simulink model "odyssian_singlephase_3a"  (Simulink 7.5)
settings: Solver=ode23t  StartTime=0.0  StopTime=10  RelTol=1e-6
undefined symbols (not defined in the file or in its folder): dfilt, DiscIntNeverNeededParam
libraries: powerlib x61, powerlib_extras x25, simulink x12, dsparch4 x2
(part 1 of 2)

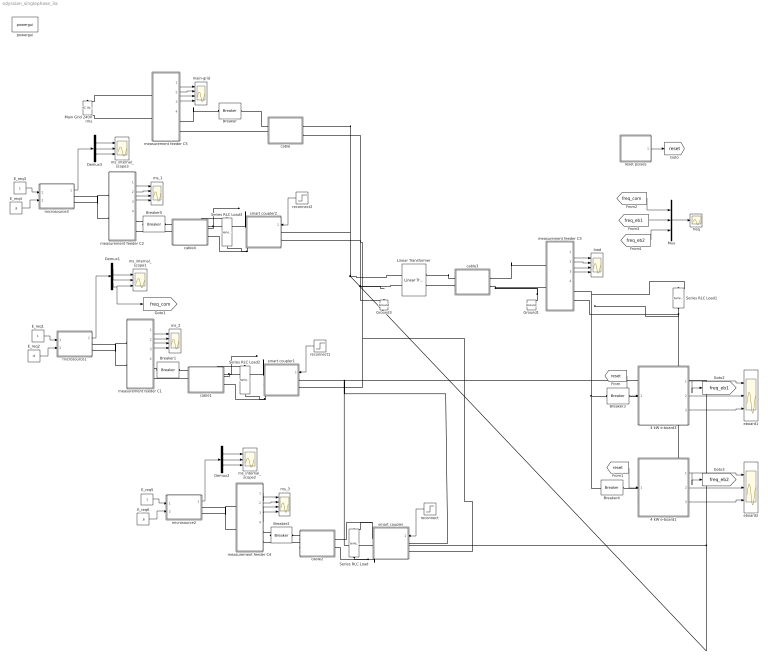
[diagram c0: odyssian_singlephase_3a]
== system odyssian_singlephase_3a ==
  " load" : Scope  NumInputPorts=4
  " main-grid" : Scope  NumInputPorts=4
  " ms_1" : Scope  NumInputPorts=4
  " ms_2" : Scope  NumInputPorts=4
  " ms_3" : Scope  NumInputPorts=4
  4 kW e-board1 : Subsystem  mask{tf=100, p=2}
      mask prompts: tf "fault_time"; p "load priority"
  4 kW e-board3 : Subsystem  mask{tf=100, p=2}
      mask prompts: tf "fault_time"; p "load priority"
  Breaker : powerlib/Elements/Breaker  DialogController=POWERSYS.PowerSysDialog  SystemSampleTime=-1  BreakerResistance=0.01  InitialState=1  SnubberResistance=1e6  SnubberCapacitance=inf  SwitchingTimes=[5]  External=off  Measurements=None  MoreParameters=off  NoBreakLoop=off
  Breaker{1..5} (5 alike) : powerlib/Elements/Breaker  DialogController=POWERSYS.PowerSysDialog  SystemSampleTime=-1  BreakerResistance=0.01  InitialState=1  SnubberResistance=1e6  SnubberCapacitance=inf  SwitchingTimes=[100]  External=off  Measurements=None  MoreParameters=off  NoBreakLoop=off
  Demux1 : Demux  Outputs=3
  Demux2 : Demux  Outputs=3
  Demux3 : Demux  Outputs=3
  E_req1 : Constant  OutDataType=fixdt(1, 16)  OutScaling=2^0
  E_req2 : Constant  Value=.8  OutDataType=fixdt(1, 16)  OutScaling=2^0
  E_req3 : Constant  OutDataType=fixdt(1, 16)  OutScaling=2^0
  E_req4 : Constant  Value=.8  OutDataType=fixdt(1, 16)  OutScaling=2^0
  E_req5 : Constant  OutDataType=fixdt(1, 16)  OutScaling=2^0
  E_req6 : Constant  Value=.8  OutDataType=fixdt(1, 16)  OutScaling=2^0
  Ground1 : powerlib/Elements/Ground  DialogController=POWERSYS.PowerSysDialog  PhysicalDomain=powersysdomain  SubClassName=unknown  LeftPortType=p1  RightPortType=p1  LConnTagsString=a
  Ground3 : powerlib/Elements/Ground  DialogController=POWERSYS.PowerSysDialog  PhysicalDomain=powersysdomain  SubClassName=unknown  LeftPortType=p1  RightPortType=p1  LConnTagsString=a
  Linear Transformer : powerlib/Elements/Linear Transformer  DialogController=POWERSYS.PowerSysDialog  PhysicalDomain=powersysdomain  SubClassName=unknown  LeftPortType=p1  RightPortType=p1  LConnTagsString=a|b  RConnTagsString=A|B  UNITS=SI  NominalPower=[ 45e3 , 60 ]  winding1=[240 0.001 1.e-5]  winding2=[120 .001 1.e-5]  ThreeWindings=off  winding3=[3.15e+05 0.7938 0.084225]  RmLm=[1.0804e+06 2866]  Measurements=All voltages and currents  DataType=on
  Main Grid 240V rms : powerlib/Electrical Sources/AC Voltage Source  DialogController=POWERSYS.PowerSysDialog  SystemSampleTime=-1  Amplitude=240*sqrt(2)  Phase=0  Frequency=60  SampleTime=0  Measurements=None
  Mux : Mux  Inputs=3
  Series RLC Load : powerlib/Elements/Series RLC Load  DialogController=POWERSYS.PowerSysDialog  PhysicalDomain=powersysdomain  SubClassName=unknown  LeftPortType=p1  RightPortType=p1  LConnTagsString=a  RConnTagsString=__new0  NominalVoltage=240  NominalFrequency=60  ActivePower=10  InductivePower=0  CapacitivePower=10*sin(acos(.88))  Setx0=off  InitialVoltage=0  SetiL0=off  InitialCurrent=0  Measurements=None
  Series RLC Load1 : powerlib/Elements/Series RLC Load  DialogController=POWERSYS.PowerSysDialog  PhysicalDomain=powersysdomain  SubClassName=unknown  LeftPortType=p1  RightPortType=p1  LConnTagsString=a  RConnTagsString=__new0  NominalVoltage=120  NominalFrequency=60  ActivePower=120  InductivePower=0  CapacitivePower=0  Setx0=off  InitialVoltage=0  SetiL0=off  InitialCurrent=0  Measurements=None
  Series RLC Load2 : powerlib/Elements/Series RLC Load  DialogController=POWERSYS.PowerSysDialog  PhysicalDomain=powersysdomain  SubClassName=unknown  LeftPortType=p1  RightPortType=p1  LConnTagsString=a  RConnTagsString=__new0  NominalVoltage=240  NominalFrequency=60  ActivePower=10  InductivePower=0  CapacitivePower=10*sin(acos(.88))  Setx0=off  InitialVoltage=0  SetiL0=off  InitialCurrent=0  Measurements=None
  Series RLC Load3 : powerlib/Elements/Series RLC Load  DialogController=POWERSYS.PowerSysDialog  PhysicalDomain=powersysdomain  SubClassName=unknown  LeftPortType=p1  RightPortType=p1  LConnTagsString=a  RConnTagsString=__new0  NominalVoltage=240  NominalFrequency=60  ActivePower=10  InductivePower=0  CapacitivePower=10*sin(acos(.88))  Setx0=off  InitialVoltage=0  SetiL0=off  InitialCurrent=0  Measurements=None
  cable : Subsystem
  cable1 : Subsystem
  cable2 : Subsystem
  cable3 : Subsystem
  cable4 : Subsystem
  eboard1 : Scope  NumInputPorts=3
  eboard2 : Scope  NumInputPorts=3
  freq : Scope
  measurement feeder C1 : Subsystem
  measurement feeder C2 : Subsystem
  measurement feeder C3 : Subsystem
  measurement feeder C4 : Subsystem
  measurement feeder C5 : Subsystem
  microsource1 : Subsystem  AncestorBlock=|
      | UWM_blocks/inverter-based
      | DG (simplified)
      | 208V - 15kVA
  microsource2 : Subsystem  AncestorBlock=|
      | UWM_blocks/inverter-based
      | DG (simplified)
      | 208V - 15kVA
  microsource3 : Subsystem  AncestorBlock=|
      | UWM_blocks/inverter-based
      | DG (simplified)
      | 208V - 15kVA
  ms_internal_scope1 : Scope  NumInputPorts=3
  ms_internal_scope2 : Scope  NumInputPorts=3
  ms_internal_scope3 : Scope  NumInputPorts=3
  powergui : powerlib/powergui  Priority=1  SystemSampleTime=-1  SimulationMode=Discrete  SampleTime=50e-5  frequency=60  SPID=off  DisableSnubberDevices=off  DisableRonSwitches=off  DisableVfSwitches=off  SwTol=0  Interpol=off  frequencyindice=0  echomessages=off  HookPort=off  DisplayEquations=off  FunctionMessages=off  EnableUseOfTLC=off  x0status=blocks  RestoreLinks=warning  ResistiveCurrentMeasurement=off  Frange=[0:2:500]  Ylog=off  Xlog=on  ShowGrid=off  save=off  variable=ZData  ZoomFFT=on  StartTime=0.0  cycles=1  DisplayStyle=1  fundamental=60  FreqAxis=off  MaxFrequency=1000  frequencyindicesteady=1  RmsSteady=1  display=off  Ts=0  methode=off
  reconnect : Step  Time=.1  SampleTime=0
  reconnect1 : Step  Time=.1  SampleTime=0
  reconnect2 : Step  Time=.1  SampleTime=0
  reset pulses : Subsystem  mask{tpulse=[50 100]}
  smart coupler : Subsystem
  smart coupler1 : Subsystem
  smart coupler2 : Subsystem
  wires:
  measurement feeder C3/1(Vm) -> " load"/1
  measurement feeder C3/2(Im) -> " load"/2
  measurement feeder C3/3(PQ) -> " load"/3
  measurement feeder C3/4(RMS (V-I)) -> " load"/4
  measurement feeder C4/1(Vm) -> " ms_3"/1
  measurement feeder C4/2(Im) -> " ms_3"/2
  measurement feeder C4/3(PQ) -> " ms_3"/3
  measurement feeder C4/4(RMS (V-I)) -> " ms_3"/4
  E_req6/1 -> microsource2/2(P_req)
  E_req5/1 -> microsource2/1(E_req)
  Demux2/2 -> ms_internal_scope2/2
  Demux2/1 -> ms_internal_scope2/1
  Demux2/3 -> ms_internal_scope2/3
  microsource2/1(m) -> Demux2/1
  reconnect/1 -> smart coupler/1(switch)
  4 kW e-board3/1(w) -> eboard1/1, [freq_eb1]
  4 kW e-board3/2(Irms) -> eboard1/2
  4 kW e-board3/3(Vrms) -> eboard1/3
  [reset] -> 4 kW e-board3/1(reset)
  4 kW e-board1/1(w) -> eboard2/1, [freq_eb2]
  4 kW e-board1/2(Irms) -> eboard2/2
  4 kW e-board1/3(Vrms) -> eboard2/3
  [reset] -> 4 kW e-board1/1(reset)
  Mux/1 -> freq/1
  reset pulses/1(Out1) -> [reset]
  [freq_com] -> Mux/1
  [freq_eb1] -> Mux/2
  [freq_eb2] -> Mux/3
  measurement feeder C5/1(Vm) -> " main-grid"/1
  measurement feeder C5/2(Im) -> " main-grid"/2
  measurement feeder C5/3(PQ) -> " main-grid"/3
  measurement feeder C5/4(RMS (V-I)) -> " main-grid"/4
  measurement feeder C1/1(Vm) -> " ms_2"/1
  measurement feeder C1/2(Im) -> " ms_2"/2
  measurement feeder C1/3(PQ) -> " ms_2"/3
  measurement feeder C1/4(RMS (V-I)) -> " ms_2"/4
  E_req2/1 -> microsource1/2(P_req)
  E_req1/1 -> microsource1/1(E_req)
  Demux1/2 -> ms_internal_scope1/2
  Demux1/1 -> ms_internal_scope1/1
  Demux1/3 -> ms_internal_scope1/3, [freq_com]
  microsource1/1(m) -> Demux1/1
  reconnect1/1 -> smart coupler1/1(switch)
  measurement feeder C2/1(Vm) -> " ms_1"/1
  measurement feeder C2/2(Im) -> " ms_1"/2
  measurement feeder C2/3(PQ) -> " ms_1"/3
  measurement feeder C2/4(RMS (V-I)) -> " ms_1"/4
  E_req4/1 -> microsource3/2(P_req)
  E_req3/1 -> microsource3/1(E_req)
  Demux3/2 -> ms_internal_scope3/2
  Demux3/1 -> ms_internal_scope3/1
  Demux3/3 -> ms_internal_scope3/3
  microsource3/1(m) -> Demux3/1
  reconnect2/1 -> smart coupler2/1(switch)
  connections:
  Breaker3/RConn1 -- measurement feeder C3/RConn1 -- Series RLC Load1/LConn1 -- Breaker4/RConn1
  Series RLC Load1/RConn1 -- measurement feeder C3/RConn2 -- 4 kW e-board3/LConn2 -- 4 kW e-board1/LConn2
  cable3/LConn2 -- Ground1/LConn1 -- measurement feeder C3/LConn2
  measurement feeder C4/LConn2 -- microsource2/RConn2
  measurement feeder C4/LConn1 -- microsource2/RConn1
  Breaker2/RConn1 -- measurement feeder C4/RConn1
  4 kW e-board3/LConn1 -- Breaker3/LConn1
  4 kW e-board1/LConn1 -- Breaker4/LConn1
  measurement feeder C5/RConn1 -- Breaker/LConn1
  cable/RConn2 -- measurement feeder C5/RConn2
  cable/RConn1 -- Breaker/RConn1
  Linear Transformer/LConn1 -- smart coupler/LConn1 -- smart coupler1/LConn1 -- cable/LConn1 -- smart coupler2/LConn1
  Linear Transformer/LConn2 -- Ground3/LConn1 -- smart coupler/LConn2 -- smart coupler1/LConn2 -- cable/LConn2 -- smart coupler2/LConn2
  cable2/RConn1 -- Breaker2/LConn1
  cable2/RConn2 -- measurement feeder C4/RConn2
  cable3/LConn1 -- measurement feeder C3/LConn1
  cable3/RConn2 -- Linear Transformer/RConn2
  cable3/RConn1 -- Linear Transformer/RConn1
  Series RLC Load/RConn1 -- cable2/LConn2 -- smart coupler/RConn2
  smart coupler/RConn1 -- Series RLC Load/LConn1 -- cable2/LConn1
  measurement feeder C5/LConn1 -- Main Grid 240V rms/RConn1
  measurement feeder C5/LConn2 -- Main Grid 240V rms/LConn1
  smart coupler1/RConn2 -- Series RLC Load2/RConn1 -- cable1/LConn2
  cable1/LConn1 -- smart coupler1/RConn1 -- Series RLC Load2/LConn1
  cable1/RConn2 -- measurement feeder C1/RConn2
  measurement feeder C1/LConn1 -- microsource1/RConn1
  cable1/RConn1 -- Breaker1/LConn1
  measurement feeder C1/LConn2 -- microsource1/RConn2
  Breaker1/RConn1 -- measurement feeder C1/RConn1
  smart coupler2/RConn2 -- Series RLC Load3/RConn1 -- cable4/LConn2
  cable4/LConn1 -- smart coupler2/RConn1 -- Series RLC Load3/LConn1
  measurement feeder C2/LConn1 -- microsource3/RConn1
  cable4/RConn2 -- measurement feeder C2/RConn2
  measurement feeder C2/LConn2 -- microsource3/RConn2
  Breaker5/RConn1 -- measurement feeder C2/RConn1
  cable4/RConn1 -- Breaker5/LConn1

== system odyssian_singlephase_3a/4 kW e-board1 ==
  reset : Inport
  Breaker : powerlib/Elements/Breaker  DialogController=POWERSYS.PowerSysDialog  SystemSampleTime=-1  BreakerResistance=0.01  InitialState=1  SnubberResistance=1e6  SnubberCapacitance=inf  SwitchingTimes="[ 1/60  5/60 ]"  External=on  Measurements=None  MoreParameters=off  NoBreakLoop=off
  Current Measurement : powerlib/Measurements/Current Measurement  DialogController=POWERSYS.PowerSysDialog  SystemSampleTime=-1  PhasorSimulation=off  OutputType=Complex  PSBequivalent=0
  Ground : powerlib/Elements/Ground  DialogController=POWERSYS.PowerSysDialog  PhysicalDomain=powersysdomain  SubClassName=unknown  LeftPortType=p1  RightPortType=p1  LConnTagsString=a
  Series RLC Load : powerlib/Elements/Series RLC Load  DialogController=POWERSYS.PowerSysDialog  PhysicalDomain=powersysdomain  SubClassName=unknown  LeftPortType=p1  RightPortType=p1  LConnTagsString=a  RConnTagsString=__new0  NominalVoltage=120  NominalFrequency=60  ActivePower=120  InductivePower=0  CapacitivePower=0  Setx0=off  InitialVoltage=0  SetiL0=off  InitialCurrent=0  Measurements=None
  Voltage  Measurement : powerlib/Measurements/Voltage Measurement  DialogController=POWERSYS.PowerSysDialog  SystemSampleTime=-1  PhasorSimulation=off  OutputType=Complex  PSBequivalent=0
  trip : Subsystem  mask{p=p}
      mask prompts: p "priority level"
  A : PMIOPort  Port=1  Side=Left
  C : PMIOPort  Port=2  Side=Left
  w : Outport  OutDataType=fixdt(1, 16)  OutScaling=2^0
  Irms : Outport  Port=2  OutDataType=fixdt(1, 16)  OutScaling=2^0
  Vrms : Outport  Port=3  OutDataType=fixdt(1, 16)  OutScaling=2^0
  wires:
  trip/1(w) -> w/1
  Current Measurement/1 -> trip/3(I)
  Voltage  Measurement/1 -> trip/2(V)
  reset/1 -> trip/1(Reset)
  trip/2(trip) -> Breaker/1
  trip/3(Irms) -> Irms/1
  trip/4(Vrms) -> Vrms/1
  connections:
  A/RConn1 -- Current Measurement/LConn1 -- Voltage  Measurement/LConn1
  Voltage  Measurement/LConn2 -- Ground/LConn1
  Current Measurement/RConn1 -- Breaker/LConn1
  Series RLC Load/LConn1 -- Breaker/RConn1
  Series RLC Load/RConn1 -- C/RConn1

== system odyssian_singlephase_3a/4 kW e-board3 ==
  reset : Inport
  Breaker : powerlib/Elements/Breaker  DialogController=POWERSYS.PowerSysDialog  SystemSampleTime=-1  BreakerResistance=0.01  InitialState=1  SnubberResistance=1e6  SnubberCapacitance=inf  SwitchingTimes="[ 1/60  5/60 ]"  External=on  Measurements=None  MoreParameters=off  NoBreakLoop=off
  Current Measurement : powerlib/Measurements/Current Measurement  DialogController=POWERSYS.PowerSysDialog  SystemSampleTime=-1  PhasorSimulation=off  OutputType=Complex  PSBequivalent=0
  Ground : powerlib/Elements/Ground  DialogController=POWERSYS.PowerSysDialog  PhysicalDomain=powersysdomain  SubClassName=unknown  LeftPortType=p1  RightPortType=p1  LConnTagsString=a
  Series RLC Load : powerlib/Elements/Series RLC Load  DialogController=POWERSYS.PowerSysDialog  PhysicalDomain=powersysdomain  SubClassName=unknown  LeftPortType=p1  RightPortType=p1  LConnTagsString=a  RConnTagsString=__new0  NominalVoltage=120  NominalFrequency=60  ActivePower=120  InductivePower=0  CapacitivePower=0  Setx0=off  InitialVoltage=0  SetiL0=off  InitialCurrent=0  Measurements=None
  Voltage  Measurement : powerlib/Measurements/Voltage Measurement  DialogController=POWERSYS.PowerSysDialog  SystemSampleTime=-1  PhasorSimulation=off  OutputType=Complex  PSBequivalent=0
  trip : Subsystem  mask{p=p}
      mask prompts: p "priority level"
  A : PMIOPort  Port=1  Side=Left
  C : PMIOPort  Port=2  Side=Left
  w : Outport  OutDataType=fixdt(1, 16)  OutScaling=2^0
  Irms : Outport  Port=2  OutDataType=fixdt(1, 16)  OutScaling=2^0
  Vrms : Outport  Port=3  OutDataType=fixdt(1, 16)  OutScaling=2^0
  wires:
  trip/1(w) -> w/1
  Current Measurement/1 -> trip/3(I)
  Voltage  Measurement/1 -> trip/2(V)
  reset/1 -> trip/1(Reset)
  trip/2(trip) -> Breaker/1
  trip/3(Irms) -> Irms/1
  trip/4(Vrms) -> Vrms/1
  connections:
  A/RConn1 -- Current Measurement/LConn1 -- Voltage  Measurement/LConn1
  Voltage  Measurement/LConn2 -- Ground/LConn1
  Current Measurement/RConn1 -- Breaker/LConn1
  Series RLC Load/LConn1 -- Breaker/RConn1
  Series RLC Load/RConn1 -- C/RConn1

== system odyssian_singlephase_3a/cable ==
  Series RLC Branch : powerlib/Elements/Series RLC Branch  DialogController=POWERSYS.PowerSysDialog  PhysicalDomain=powersysdomain  SubClassName=unknown  LeftPortType=p1  RightPortType=p1  LConnTagsString=__new0  RConnTagsString=__new0  BranchType=RL  Resistance=.001  Inductance=1.e-5  SetiL0=off  InitialCurrent=0  Capacitance=1e-6  Setx0=off  InitialVoltage=0  Measurements=None
  A : PMIOPort  Tag=PMCPort  Port=1  Side=Left
  A' : PMIOPort  Tag=PMCPort  Port=2  Side=Right
  B' : PMIOPort  Tag=PMCPort  Port=3  Side=Right
  B : PMIOPort  Tag=PMCPort  Port=4  Side=Left
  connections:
  A/RConn1 -- Series RLC Branch/LConn1
  A'/RConn1 -- Series RLC Branch/RConn1
  B/RConn1 -- B'/RConn1

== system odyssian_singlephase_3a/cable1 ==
  Series RLC Branch : powerlib/Elements/Series RLC Branch  DialogController=POWERSYS.PowerSysDialog  PhysicalDomain=powersysdomain  SubClassName=unknown  LeftPortType=p1  RightPortType=p1  LConnTagsString=__new0  RConnTagsString=__new0  BranchType=RL  Resistance=.001  Inductance=1.e-6  SetiL0=off  InitialCurrent=0  Capacitance=1e-6  Setx0=off  InitialVoltage=0  Measurements=None
  A : PMIOPort  Tag=PMCPort  Port=1  Side=Left
  A' : PMIOPort  Tag=PMCPort  Port=2  Side=Right
  B' : PMIOPort  Tag=PMCPort  Port=3  Side=Right
  B : PMIOPort  Tag=PMCPort  Port=4  Side=Left
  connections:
  A/RConn1 -- Series RLC Branch/LConn1
  Series RLC Branch/RConn1 -- A'/RConn1
  B/RConn1 -- B'/RConn1

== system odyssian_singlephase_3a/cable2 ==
  Series RLC Branch : powerlib/Elements/Series RLC Branch  DialogController=POWERSYS.PowerSysDialog  PhysicalDomain=powersysdomain  SubClassName=unknown  LeftPortType=p1  RightPortType=p1  LConnTagsString=__new0  RConnTagsString=__new0  BranchType=RL  Resistance=.001  Inductance=1.e-6  SetiL0=off  InitialCurrent=0  Capacitance=1e-6  Setx0=off  InitialVoltage=0  Measurements=None
  A : PMIOPort  Tag=PMCPort  Port=1  Side=Left
  A' : PMIOPort  Tag=PMCPort  Port=2  Side=Right
  B' : PMIOPort  Tag=PMCPort  Port=3  Side=Right
  B : PMIOPort  Tag=PMCPort  Port=4  Side=Left
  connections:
  A/RConn1 -- Series RLC Branch/LConn1
  Series RLC Branch/RConn1 -- A'/RConn1
  B/RConn1 -- B'/RConn1

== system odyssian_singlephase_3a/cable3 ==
  Series RLC Branch : powerlib/Elements/Series RLC Branch  DialogController=POWERSYS.PowerSysDialog  PhysicalDomain=powersysdomain  SubClassName=unknown  LeftPortType=p1  RightPortType=p1  LConnTagsString=__new0  RConnTagsString=__new0  BranchType=RL  Resistance=.001  Inductance=1.e-6  SetiL0=off  InitialCurrent=0  Capacitance=1e-6  Setx0=off  InitialVoltage=0  Measurements=None
  A : PMIOPort  Tag=PMCPort  Port=1  Side=Left
  A' : PMIOPort  Tag=PMCPort  Port=2  Side=Right
  B' : PMIOPort  Tag=PMCPort  Port=3  Side=Right
  B : PMIOPort  Tag=PMCPort  Port=4  Side=Left
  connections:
  A/RConn1 -- Series RLC Branch/LConn1
  Series RLC Branch/RConn1 -- A'/RConn1
  B/RConn1 -- B'/RConn1

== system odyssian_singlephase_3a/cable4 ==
  Series RLC Branch : powerlib/Elements/Series RLC Branch  DialogController=POWERSYS.PowerSysDialog  PhysicalDomain=powersysdomain  SubClassName=unknown  LeftPortType=p1  RightPortType=p1  LConnTagsString=__new0  RConnTagsString=__new0  BranchType=RL  Resistance=.001  Inductance=1.e-6  SetiL0=off  InitialCurrent=0  Capacitance=1e-6  Setx0=off  InitialVoltage=0  Measurements=None
  A : PMIOPort  Tag=PMCPort  Port=1  Side=Left
  A' : PMIOPort  Tag=PMCPort  Port=2  Side=Right
  B' : PMIOPort  Tag=PMCPort  Port=3  Side=Right
  B : PMIOPort  Tag=PMCPort  Port=4  Side=Left
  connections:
  A/RConn1 -- Series RLC Branch/LConn1
  Series RLC Branch/RConn1 -- A'/RConn1
  B/RConn1 -- B'/RConn1

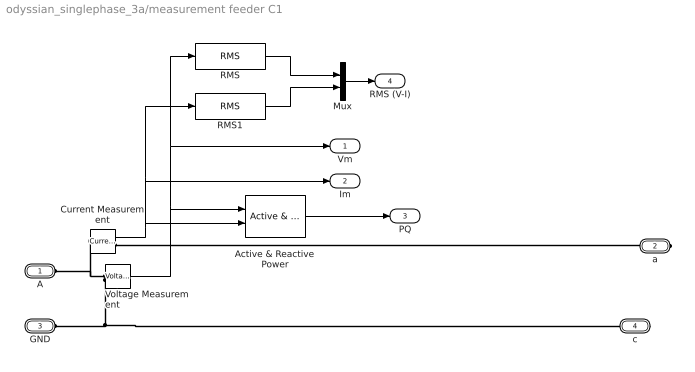
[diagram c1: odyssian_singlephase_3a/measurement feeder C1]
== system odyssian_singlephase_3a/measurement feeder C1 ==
  Active & Reactive Power : powerlib_extras/Measurements/Active & Reactive Power  DialogController=POWERSYS.PowerSysDialog  SystemSampleTime=-1  f1=60
  Current Measurement : powerlib/Measurements/Current Measurement  DialogController=POWERSYS.PowerSysDialog  SystemSampleTime=-1  PhasorSimulation=off  OutputType=Complex  PSBequivalent=0
  Mux : Mux  Inputs=2
  RMS : powerlib_extras/Measurements/RMS  DialogController=POWERSYS.PowerSysDialog  SystemSampleTime=-1  f1=60
  RMS1 : powerlib_extras/Measurements/RMS  DialogController=POWERSYS.PowerSysDialog  SystemSampleTime=-1  f1=60
  Voltage Measurement : powerlib/Measurements/Voltage Measurement  DialogController=POWERSYS.PowerSysDialog  SystemSampleTime=-1  PhasorSimulation=off  OutputType=Complex  PSBequivalent=0
  A : PMIOPort  Port=1  Side=Left
  a : PMIOPort  Port=2  Side=Right
  GND : PMIOPort  Port=3  Side=Left
  c : PMIOPort  Port=4  Side=Right
  Vm : Outport  OutDataType=fixdt(1, 16)  OutScaling=2^0
  Im : Outport  Port=2  OutDataType=fixdt(1, 16)  OutScaling=2^0
  PQ : Outport  Port=3  OutDataType=fixdt(1, 16)  OutScaling=2^0
  RMS (V-I) : Outport  Port=4  OutDataType=fixdt(1, 16)  OutScaling=2^0
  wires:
  Mux/1 -> RMS (V-I)/1
  Current Measurement/1 -> Im/1, RMS1/1, Active & Reactive Power/2
  Voltage Measurement/1 -> Vm/1, RMS/1, Active & Reactive Power/1
  Active & Reactive Power/1 -> PQ/1
  RMS/1 -> Mux/1
  RMS1/1 -> Mux/2
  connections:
  a/RConn1 -- Current Measurement/RConn1
  Voltage Measurement/LConn1 -- A/RConn1 -- Current Measurement/LConn1
  Voltage Measurement/LConn2 -- GND/RConn1 -- c/RConn1

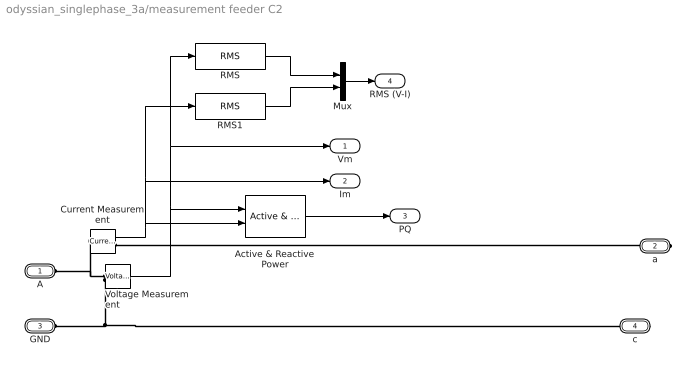
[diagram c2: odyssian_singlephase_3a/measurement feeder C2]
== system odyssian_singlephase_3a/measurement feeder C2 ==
  Active & Reactive Power : powerlib_extras/Measurements/Active & Reactive Power  DialogController=POWERSYS.PowerSysDialog  SystemSampleTime=-1  f1=60
  Current Measurement : powerlib/Measurements/Current Measurement  DialogController=POWERSYS.PowerSysDialog  SystemSampleTime=-1  PhasorSimulation=off  OutputType=Complex  PSBequivalent=0
  Mux : Mux  Inputs=2
  RMS : powerlib_extras/Measurements/RMS  DialogController=POWERSYS.PowerSysDialog  SystemSampleTime=-1  f1=60
  RMS1 : powerlib_extras/Measurements/RMS  DialogController=POWERSYS.PowerSysDialog  SystemSampleTime=-1  f1=60
  Voltage Measurement : powerlib/Measurements/Voltage Measurement  DialogController=POWERSYS.PowerSysDialog  SystemSampleTime=-1  PhasorSimulation=off  OutputType=Complex  PSBequivalent=0
  A : PMIOPort  Port=1  Side=Left
  a : PMIOPort  Port=2  Side=Right
  GND : PMIOPort  Port=3  Side=Left
  c : PMIOPort  Port=4  Side=Right
  Vm : Outport  OutDataType=fixdt(1, 16)  OutScaling=2^0
  Im : Outport  Port=2  OutDataType=fixdt(1, 16)  OutScaling=2^0
  PQ : Outport  Port=3  OutDataType=fixdt(1, 16)  OutScaling=2^0
  RMS (V-I) : Outport  Port=4  OutDataType=fixdt(1, 16)  OutScaling=2^0
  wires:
  Mux/1 -> RMS (V-I)/1
  Current Measurement/1 -> Im/1, RMS1/1, Active & Reactive Power/2
  Voltage Measurement/1 -> Vm/1, RMS/1, Active & Reactive Power/1
  Active & Reactive Power/1 -> PQ/1
  RMS/1 -> Mux/1
  RMS1/1 -> Mux/2
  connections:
  a/RConn1 -- Current Measurement/RConn1
  Voltage Measurement/LConn1 -- A/RConn1 -- Current Measurement/LConn1
  Voltage Measurement/LConn2 -- GND/RConn1 -- c/RConn1

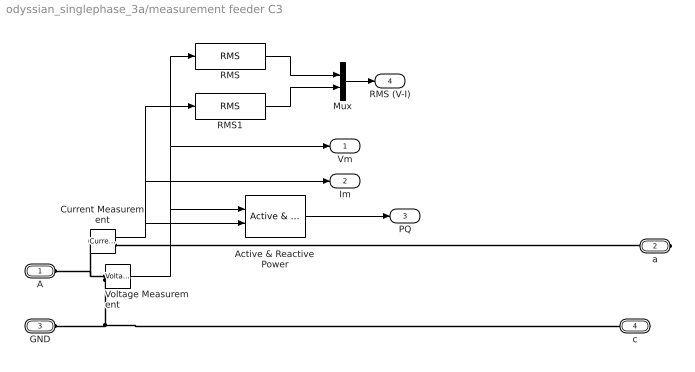
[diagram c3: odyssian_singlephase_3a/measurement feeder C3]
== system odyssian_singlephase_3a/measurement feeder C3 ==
  Active & Reactive Power : powerlib_extras/Measurements/Active & Reactive Power  DialogController=POWERSYS.PowerSysDialog  SystemSampleTime=-1  f1=60
  Current Measurement : powerlib/Measurements/Current Measurement  DialogController=POWERSYS.PowerSysDialog  SystemSampleTime=-1  PhasorSimulation=off  OutputType=Complex  PSBequivalent=0
  Mux : Mux  Inputs=2
  RMS : powerlib_extras/Measurements/RMS  DialogController=POWERSYS.PowerSysDialog  SystemSampleTime=-1  f1=60
  RMS1 : powerlib_extras/Measurements/RMS  DialogController=POWERSYS.PowerSysDialog  SystemSampleTime=-1  f1=60
  Voltage Measurement : powerlib/Measurements/Voltage Measurement  DialogController=POWERSYS.PowerSysDialog  SystemSampleTime=-1  PhasorSimulation=off  OutputType=Complex  PSBequivalent=0
  A : PMIOPort  Port=1  Side=Left
  a : PMIOPort  Port=2  Side=Right
  GND : PMIOPort  Port=3  Side=Left
  c : PMIOPort  Port=4  Side=Right
  Vm : Outport  OutDataType=fixdt(1, 16)  OutScaling=2^0
  Im : Outport  Port=2  OutDataType=fixdt(1, 16)  OutScaling=2^0
  PQ : Outport  Port=3  OutDataType=fixdt(1, 16)  OutScaling=2^0
  RMS (V-I) : Outport  Port=4  OutDataType=fixdt(1, 16)  OutScaling=2^0
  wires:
  Mux/1 -> RMS (V-I)/1
  Current Measurement/1 -> Im/1, RMS1/1, Active & Reactive Power/2
  Voltage Measurement/1 -> Vm/1, RMS/1, Active & Reactive Power/1
  Active & Reactive Power/1 -> PQ/1
  RMS/1 -> Mux/1
  RMS1/1 -> Mux/2
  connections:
  a/RConn1 -- Current Measurement/RConn1
  Voltage Measurement/LConn1 -- A/RConn1 -- Current Measurement/LConn1
  Voltage Measurement/LConn2 -- GND/RConn1 -- c/RConn1

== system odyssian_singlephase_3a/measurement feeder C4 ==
  Active & Reactive Power : powerlib_extras/Measurements/Active & Reactive Power  DialogController=POWERSYS.PowerSysDialog  SystemSampleTime=-1  f1=60
  Current Measurement : powerlib/Measurements/Current Measurement  DialogController=POWERSYS.PowerSysDialog  SystemSampleTime=-1  PhasorSimulation=off  OutputType=Complex  PSBequivalent=0
  Mux : Mux  Inputs=2
  RMS : powerlib_extras/Measurements/RMS  DialogController=POWERSYS.PowerSysDialog  SystemSampleTime=-1  f1=60
  RMS1 : powerlib_extras/Measurements/RMS  DialogController=POWERSYS.PowerSysDialog  SystemSampleTime=-1  f1=60
  Voltage Measurement : powerlib/Measurements/Voltage Measurement  DialogController=POWERSYS.PowerSysDialog  SystemSampleTime=-1  PhasorSimulation=off  OutputType=Complex  PSBequivalent=0
  A : PMIOPort  Port=1  Side=Left
  a : PMIOPort  Port=2  Side=Right
  GND : PMIOPort  Port=3  Side=Left
  c : PMIOPort  Port=4  Side=Right
  Vm : Outport  OutDataType=fixdt(1, 16)  OutScaling=2^0
  Im : Outport  Port=2  OutDataType=fixdt(1, 16)  OutScaling=2^0
  PQ : Outport  Port=3  OutDataType=fixdt(1, 16)  OutScaling=2^0
  RMS (V-I) : Outport  Port=4  OutDataType=fixdt(1, 16)  OutScaling=2^0
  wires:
  Mux/1 -> RMS (V-I)/1
  Current Measurement/1 -> Im/1, RMS1/1, Active & Reactive Power/2
  Voltage Measurement/1 -> Vm/1, RMS/1, Active & Reactive Power/1
  Active & Reactive Power/1 -> PQ/1
  RMS/1 -> Mux/1
  RMS1/1 -> Mux/2
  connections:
  a/RConn1 -- Current Measurement/RConn1
  Voltage Measurement/LConn1 -- A/RConn1 -- Current Measurement/LConn1
  Voltage Measurement/LConn2 -- GND/RConn1 -- c/RConn1

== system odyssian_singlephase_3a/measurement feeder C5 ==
  Active & Reactive Power : powerlib_extras/Measurements/Active & Reactive Power  DialogController=POWERSYS.PowerSysDialog  SystemSampleTime=-1  f1=60
  Current Measurement : powerlib/Measurements/Current Measurement  DialogController=POWERSYS.PowerSysDialog  SystemSampleTime=-1  PhasorSimulation=off  OutputType=Complex  PSBequivalent=0
  Mux : Mux  Inputs=2
  RMS : powerlib_extras/Measurements/RMS  DialogController=POWERSYS.PowerSysDialog  SystemSampleTime=-1  f1=60
  RMS1 : powerlib_extras/Measurements/RMS  DialogController=POWERSYS.PowerSysDialog  SystemSampleTime=-1  f1=60
  Voltage Measurement : powerlib/Measurements/Voltage Measurement  DialogController=POWERSYS.PowerSysDialog  SystemSampleTime=-1  PhasorSimulation=off  OutputType=Complex  PSBequivalent=0
  A : PMIOPort  Port=1  Side=Left
  a : PMIOPort  Port=2  Side=Right
  GND : PMIOPort  Port=3  Side=Left
  c : PMIOPort  Port=4  Side=Right
  Vm : Outport  OutDataType=fixdt(1, 16)  OutScaling=2^0
  Im : Outport  Port=2  OutDataType=fixdt(1, 16)  OutScaling=2^0
  PQ : Outport  Port=3  OutDataType=fixdt(1, 16)  OutScaling=2^0
  RMS (V-I) : Outport  Port=4  OutDataType=fixdt(1, 16)  OutScaling=2^0
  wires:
  Mux/1 -> RMS (V-I)/1
  Current Measurement/1 -> Im/1, RMS1/1, Active & Reactive Power/2
  Voltage Measurement/1 -> Vm/1, RMS/1, Active & Reactive Power/1
  Active & Reactive Power/1 -> PQ/1
  RMS/1 -> Mux/1
  RMS1/1 -> Mux/2
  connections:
  a/RConn1 -- Current Measurement/RConn1
  Voltage Measurement/LConn1 -- A/RConn1 -- Current Measurement/LConn1
  Voltage Measurement/LConn2 -- GND/RConn1 -- c/RConn1

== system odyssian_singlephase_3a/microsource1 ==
  E_req : Inport
  P_req : Inport  Port=2
  Current Measurement : powerlib/Measurements/Current Measurement  DialogController=POWERSYS.PowerSysDialog  SystemSampleTime=-1  PhasorSimulation=off  OutputType=Complex  PSBequivalent=0
  Gain : Gain  Gain=1/(2*pi)  ParameterDataType=fixdt(1, 16)  ParameterScaling=2^0  OutDataType=fixdt(1, 16)  OutScaling=2^0
  Linear Transformer : powerlib/Elements/Linear Transformer  DialogController=POWERSYS.PowerSysDialog  PhysicalDomain=powersysdomain  SubClassName=unknown  LeftPortType=p1  RightPortType=p1  LConnTagsString=a|b  RConnTagsString=A|B  UNITS=SI  NominalPower=[ 45e3 , 60 ]  winding1=[240 0.001 1.e-5]  winding2=[240 0.001 1.e-5]  ThreeWindings=off  winding3=[3.15e+05 0.7938 0.084225]  RmLm=[1.0804e+06 2866]  Measurements=All voltages and currents  DataType=on
  Mux : Mux  Inputs=3
  Parallel RLC Branch : powerlib/Elements/Parallel RLC Branch  DialogController=POWERSYS.PowerSysDialog  PhysicalDomain=powersysdomain  SubClassName=unknown  LeftPortType=p1  RightPortType=p1  LConnTagsString=a  RConnTagsString=__new0  BranchType=L  Resistance=1  Inductance=1.e-1  SetiL0=off  InitialCurrent=0  Capacitance=1e-6  Setx0=off  InitialVoltage=0  Measurements=None
  UWM_controller : Subsystem  mask{Vbase=240*sqrt(2), Sbase=200}
  Voltage Measurement : powerlib/Measurements/Voltage Measurement  DialogController=POWERSYS.PowerSysDialog  SystemSampleTime=-1  PhasorSimulation=off  OutputType=Complex  PSBequivalent=0
  microsource : Subsystem
  a : PMIOPort  Port=1  Side=Right
  GND : PMIOPort  Port=2  Side=Right
  m : Outport  OutDataType=fixdt(1, 16)  OutScaling=2^0
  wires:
  E_req/1 -> UWM_controller/3(E_req)
  P_req/1 -> UWM_controller/4(P_req)
  UWM_controller/1(Vpk) -> microsource/1(Vpk)
  UWM_controller/2(w) -> microsource/2(w), Gain/1
  Mux/1 -> m/1
  Gain/1 -> Mux/3
  Current Measurement/1 -> Mux/2, UWM_controller/2(i_meas)
  Voltage Measurement/1 -> Mux/1, UWM_controller/1(v_meas)
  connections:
  GND/RConn1 -- Voltage Measurement/LConn2 -- Linear Transformer/RConn2
  Linear Transformer/RConn1 -- Voltage Measurement/LConn1 -- Current Measurement/LConn1
  a/RConn1 -- Current Measurement/RConn1
  Parallel RLC Branch/LConn1 -- microsource/RConn1
  Linear Transformer/LConn1 -- Parallel RLC Branch/RConn1
  Linear Transformer/LConn2 -- microsource/RConn2

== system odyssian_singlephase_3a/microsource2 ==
  E_req : Inport
  P_req : Inport  Port=2
  Current Measurement : powerlib/Measurements/Current Measurement  DialogController=POWERSYS.PowerSysDialog  SystemSampleTime=-1  PhasorSimulation=off  OutputType=Complex  PSBequivalent=0
  Gain : Gain  Gain=1/(2*pi)  ParameterDataType=fixdt(1, 16)  ParameterScaling=2^0  OutDataType=fixdt(1, 16)  OutScaling=2^0
  Linear Transformer : powerlib/Elements/Linear Transformer  DialogController=POWERSYS.PowerSysDialog  PhysicalDomain=powersysdomain  SubClassName=unknown  LeftPortType=p1  RightPortType=p1  LConnTagsString=a|b  RConnTagsString=A|B  UNITS=SI  NominalPower=[ 45e3 , 60 ]  winding1=[240 0.001 1.e-5]  winding2=[240 0.001 1.e-5]  ThreeWindings=off  winding3=[3.15e+05 0.7938 0.084225]  RmLm=[1.0804e+06 2866]  Measurements=All voltages and currents  DataType=on
  Mux : Mux  Inputs=3
  Parallel RLC Branch : powerlib/Elements/Parallel RLC Branch  DialogController=POWERSYS.PowerSysDialog  PhysicalDomain=powersysdomain  SubClassName=unknown  LeftPortType=p1  RightPortType=p1  LConnTagsString=a  RConnTagsString=__new0  BranchType=L  Resistance=1  Inductance=1.e-1  SetiL0=off  InitialCurrent=0  Capacitance=1e-6  Setx0=off  InitialVoltage=0  Measurements=None
  UWM_controller : Subsystem  mask{Vbase=240*sqrt(2), Sbase=200}
  Voltage Measurement : powerlib/Measurements/Voltage Measurement  DialogController=POWERSYS.PowerSysDialog  SystemSampleTime=-1  PhasorSimulation=off  OutputType=Complex  PSBequivalent=0
  microsource : Subsystem
  a : PMIOPort  Port=1  Side=Right
  GND : PMIOPort  Port=2  Side=Right
  m : Outport  OutDataType=fixdt(1, 16)  OutScaling=2^0
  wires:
  E_req/1 -> UWM_controller/3(E_req)
  P_req/1 -> UWM_controller/4(P_req)
  UWM_controller/1(Vpk) -> microsource/1(Vpk)
  UWM_controller/2(w) -> microsource/2(w), Gain/1
  Mux/1 -> m/1
  Gain/1 -> Mux/3
  Current Measurement/1 -> Mux/2, UWM_controller/2(i_meas)
  Voltage Measurement/1 -> Mux/1, UWM_controller/1(v_meas)
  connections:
  GND/RConn1 -- Voltage Measurement/LConn2 -- Linear Transformer/RConn2
  Linear Transformer/RConn1 -- Voltage Measurement/LConn1 -- Current Measurement/LConn1
  a/RConn1 -- Current Measurement/RConn1
  Parallel RLC Branch/LConn1 -- microsource/RConn1
  Linear Transformer/LConn1 -- Parallel RLC Branch/RConn1
  Linear Transformer/LConn2 -- microsource/RConn2

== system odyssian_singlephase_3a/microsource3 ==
  E_req : Inport
  P_req : Inport  Port=2
  Current Measurement : powerlib/Measurements/Current Measurement  DialogController=POWERSYS.PowerSysDialog  SystemSampleTime=-1  PhasorSimulation=off  OutputType=Complex  PSBequivalent=0
  Gain : Gain  Gain=1/(2*pi)  ParameterDataType=fixdt(1, 16)  ParameterScaling=2^0  OutDataType=fixdt(1, 16)  OutScaling=2^0
  Linear Transformer : powerlib/Elements/Linear Transformer  DialogController=POWERSYS.PowerSysDialog  PhysicalDomain=powersysdomain  SubClassName=unknown  LeftPortType=p1  RightPortType=p1  LConnTagsString=a|b  RConnTagsString=A|B  UNITS=SI  NominalPower=[ 45e3 , 60 ]  winding1=[240 0.001 1.e-5]  winding2=[240 0.001 1.e-5]  ThreeWindings=off  winding3=[3.15e+05 0.7938 0.084225]  RmLm=[1.0804e+06 2866]  Measurements=All voltages and currents  DataType=on
  Mux : Mux  Inputs=3
  Parallel RLC Branch : powerlib/Elements/Parallel RLC Branch  DialogController=POWERSYS.PowerSysDialog  PhysicalDomain=powersysdomain  SubClassName=unknown  LeftPortType=p1  RightPortType=p1  LConnTagsString=a  RConnTagsString=__new0  BranchType=L  Resistance=1  Inductance=1.e-1  SetiL0=off  InitialCurrent=0  Capacitance=1e-6  Setx0=off  InitialVoltage=0  Measurements=None
  UWM_controller : Subsystem  mask{Vbase=240*sqrt(2), Sbase=200}
  Voltage Measurement : powerlib/Measurements/Voltage Measurement  DialogController=POWERSYS.PowerSysDialog  SystemSampleTime=-1  PhasorSimulation=off  OutputType=Complex  PSBequivalent=0
  microsource : Subsystem
  a : PMIOPort  Port=1  Side=Right
  GND : PMIOPort  Port=2  Side=Right
  m : Outport  OutDataType=fixdt(1, 16)  OutScaling=2^0
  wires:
  E_req/1 -> UWM_controller/3(E_req)
  P_req/1 -> UWM_controller/4(P_req)
  UWM_controller/1(Vpk) -> microsource/1(Vpk)
  UWM_controller/2(w) -> microsource/2(w), Gain/1
  Mux/1 -> m/1
  Gain/1 -> Mux/3
  Current Measurement/1 -> Mux/2, UWM_controller/2(i_meas)
  Voltage Measurement/1 -> Mux/1, UWM_controller/1(v_meas)
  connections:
  GND/RConn1 -- Voltage Measurement/LConn2 -- Linear Transformer/RConn2
  Linear Transformer/RConn1 -- Voltage Measurement/LConn1 -- Current Measurement/LConn1
  a/RConn1 -- Current Measurement/RConn1
  Parallel RLC Branch/LConn1 -- microsource/RConn1
  Linear Transformer/LConn1 -- Parallel RLC Branch/RConn1
  Linear Transformer/LConn2 -- microsource/RConn2

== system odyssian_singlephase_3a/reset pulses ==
  Sum : Sum  Inputs=|++  OutDataType=fixdt(1, 16)  OutScaling=2^0
  pulse : Subsystem  mask{tstart=tpulse(1), dt=.1}
  pulse1 : Subsystem  mask{tstart=tpulse(2), dt=.1}
  Out1 : Outport
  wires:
  pulse/1(Out1) -> Sum/1
  pulse1/1(Out1) -> Sum/2
  Sum/1 -> Out1/1

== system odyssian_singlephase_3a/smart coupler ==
  switch : Inport  OutDataType=fixdt(1, 16)  OutScaling=2^0
  Abs : Abs  OutDataType=fixdt(1, 16)  OutScaling=2^0
  Breaker : powerlib/Elements/Breaker  DialogController=POWERSYS.PowerSysDialog  SystemSampleTime=-1  BreakerResistance=0.01  InitialState=0  SnubberResistance=1e6  SnubberCapacitance=inf  SwitchingTimes="[ 1/60  5/60 ]"  External=on  Measurements=None  MoreParameters=off  NoBreakLoop=off
  Level-2 M-file S-Function : M-S-Function  FunctionName=smart_coupler
  Scope : Scope  NumInputPorts=3
  Transfer Fcn : TransferFcn  Numerator=[100]  Denominator=[1 100]
  Voltage Measurement : powerlib/Measurements/Voltage Measurement  DialogController=POWERSYS.PowerSysDialog  SystemSampleTime=-1  PhasorSimulation=off  OutputType=Complex  PSBequivalent=0
  A : PMIOPort  Port=1  Side=Left
  C : PMIOPort  Port=2  Side=Left
  a : PMIOPort  Port=3  Side=Right
  c : PMIOPort  Port=4  Side=Right
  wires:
  switch/1 -> Level-2 M-file S-Function/2, Scope/2
  Level-2 M-file S-Function/1 -> Scope/1, Breaker/1
  Voltage Measurement/1 -> Abs/1
  Abs/1 -> Transfer Fcn/1
  Transfer Fcn/1 -> Level-2 M-file S-Function/1, Scope/3
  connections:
  Breaker/LConn1 -- A/RConn1 -- Voltage Measurement/LConn1
  Breaker/RConn1 -- Voltage Measurement/LConn2 -- a/RConn1
  c/RConn1 -- C/RConn1

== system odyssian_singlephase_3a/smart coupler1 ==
  switch : Inport  OutDataType=fixdt(1, 16)  OutScaling=2^0
  Abs : Abs  OutDataType=fixdt(1, 16)  OutScaling=2^0
  Breaker : powerlib/Elements/Breaker  DialogController=POWERSYS.PowerSysDialog  SystemSampleTime=-1  BreakerResistance=0.01  InitialState=0  SnubberResistance=1e6  SnubberCapacitance=inf  SwitchingTimes="[ 1/60  5/60 ]"  External=on  Measurements=None  MoreParameters=off  NoBreakLoop=off
  Level-2 M-file S-Function : M-S-Function  FunctionName=smart_coupler
  Scope : Scope  NumInputPorts=3
  Transfer Fcn : TransferFcn  Numerator=[100]  Denominator=[1 100]
  Voltage Measurement : powerlib/Measurements/Voltage Measurement  DialogController=POWERSYS.PowerSysDialog  SystemSampleTime=-1  PhasorSimulation=off  OutputType=Complex  PSBequivalent=0
  A : PMIOPort  Port=1  Side=Left
  C : PMIOPort  Port=2  Side=Left
  a : PMIOPort  Port=3  Side=Right
  c : PMIOPort  Port=4  Side=Right
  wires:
  switch/1 -> Level-2 M-file S-Function/2, Scope/2
  Level-2 M-file S-Function/1 -> Scope/1, Breaker/1
  Voltage Measurement/1 -> Abs/1
  Abs/1 -> Transfer Fcn/1
  Transfer Fcn/1 -> Level-2 M-file S-Function/1, Scope/3
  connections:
  Breaker/LConn1 -- A/RConn1 -- Voltage Measurement/LConn1
  Breaker/RConn1 -- Voltage Measurement/LConn2 -- a/RConn1
  c/RConn1 -- C/RConn1

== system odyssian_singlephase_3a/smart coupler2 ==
  switch : Inport  OutDataType=fixdt(1, 16)  OutScaling=2^0
  Abs : Abs  OutDataType=fixdt(1, 16)  OutScaling=2^0
  Breaker : powerlib/Elements/Breaker  DialogController=POWERSYS.PowerSysDialog  SystemSampleTime=-1  BreakerResistance=0.01  InitialState=0  SnubberResistance=1e6  SnubberCapacitance=inf  SwitchingTimes="[ 1/60  5/60 ]"  External=on  Measurements=None  MoreParameters=off  NoBreakLoop=off
  Level-2 M-file S-Function : M-S-Function  FunctionName=smart_coupler
  Scope : Scope  NumInputPorts=3
  Transfer Fcn : TransferFcn  Numerator=[100]  Denominator=[1 100]
  Voltage Measurement : powerlib/Measurements/Voltage Measurement  DialogController=POWERSYS.PowerSysDialog  SystemSampleTime=-1  PhasorSimulation=off  OutputType=Complex  PSBequivalent=0
  A : PMIOPort  Port=1  Side=Left
  C : PMIOPort  Port=2  Side=Left
  a : PMIOPort  Port=3  Side=Right
  c : PMIOPort  Port=4  Side=Right
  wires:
  switch/1 -> Level-2 M-file S-Function/2, Scope/2
  Level-2 M-file S-Function/1 -> Scope/1, Breaker/1
  Voltage Measurement/1 -> Abs/1
  Abs/1 -> Transfer Fcn/1
  Transfer Fcn/1 -> Level-2 M-file S-Function/1, Scope/3
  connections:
  Breaker/LConn1 -- A/RConn1 -- Voltage Measurement/LConn1
  Breaker/RConn1 -- Voltage Measurement/LConn2 -- a/RConn1
  c/RConn1 -- C/RConn1

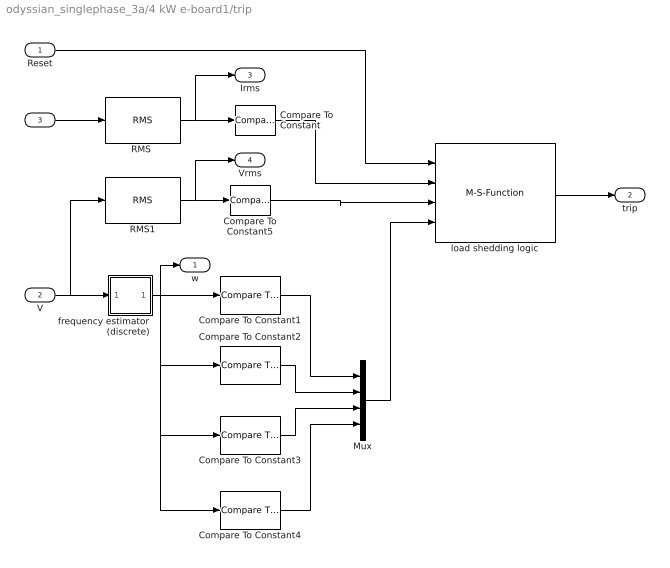
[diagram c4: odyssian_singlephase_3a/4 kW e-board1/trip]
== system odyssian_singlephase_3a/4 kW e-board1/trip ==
  Reset : Inport
  V : Inport  Port=2
  I : Inport  Port=3
  Compare To Constant : simulink/Logic and Bit Operations/Compare To Constant  SystemSampleTime=-1  relop=>=  const=100  LogicOutDataTypeMode=boolean
  Compare To Constant1 : simulink/Logic and Bit Operations/Compare To Constant  SystemSampleTime=-1  relop=<=  const=59.8  LogicOutDataTypeMode=boolean
  Compare To Constant2 : simulink/Logic and Bit Operations/Compare To Constant  SystemSampleTime=-1  relop=<=  const=59.5  LogicOutDataTypeMode=boolean
  Compare To Constant3 : simulink/Logic and Bit Operations/Compare To Constant  SystemSampleTime=-1  relop=>=  const=59.9  LogicOutDataTypeMode=boolean
  Compare To Constant4 : simulink/Logic and Bit Operations/Compare To Constant  SystemSampleTime=-1  relop=<=  const=58.6  LogicOutDataTypeMode=boolean
  Compare To Constant5 : simulink/Logic and Bit Operations/Compare To Constant  SystemSampleTime=-1  relop=<=  const=100  LogicOutDataTypeMode=boolean
  Mux : Mux
  "RMS " : powerlib_extras/Measurements/RMS  DialogController=POWERSYS.PowerSysDialog  SystemSampleTime=-1  f1=60
  RMS1 : powerlib_extras/Measurements/RMS  DialogController=POWERSYS.PowerSysDialog  SystemSampleTime=-1  f1=60
  frequency estimator (discrete) : Subsystem  mask{dt=0.010}
      mask prompts: dt "sample time"
  load shedding logic : M-S-Function  FunctionName=load_shedding_logic  Parameters=p
  w : Outport  OutDataType=fixdt(1, 16)  OutScaling=2^0
  trip : Outport  Port=2
  Irms : Outport  Port=3  OutDataType=fixdt(1, 16)  OutScaling=2^0
  Vrms : Outport  Port=4  OutDataType=fixdt(1, 16)  OutScaling=2^0
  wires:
  "RMS "/1 -> Compare To Constant/1, Irms/1
  I/1 -> "RMS "/1
  Reset/1 -> load shedding logic/1
  Compare To Constant/1 -> load shedding logic/2
  load shedding logic/1 -> trip/1
  V/1 -> frequency estimator (discrete)/1(v), RMS1/1
  frequency estimator (discrete)/1(w) -> Compare To Constant1/1, w/1, Compare To Constant2/1, Compare To Constant3/1, Compare To Constant4/1
  Compare To Constant1/1 -> Mux/1
  Compare To Constant2/1 -> Mux/2
  Compare To Constant3/1 -> Mux/3
  Compare To Constant4/1 -> Mux/4
  RMS1/1 -> Compare To Constant5/1, Vrms/1
  Compare To Constant5/1 -> load shedding logic/3
  Mux/1 -> load shedding logic/4

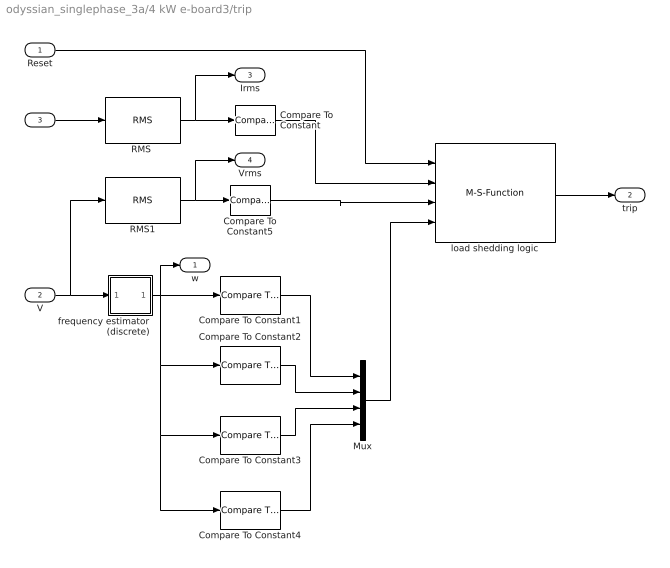
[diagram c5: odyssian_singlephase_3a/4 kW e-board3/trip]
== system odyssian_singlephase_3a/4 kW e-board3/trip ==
  Reset : Inport
  V : Inport  Port=2
  I : Inport  Port=3
  Compare To Constant : simulink/Logic and Bit Operations/Compare To Constant  SystemSampleTime=-1  relop=>=  const=100  LogicOutDataTypeMode=boolean
  Compare To Constant1 : simulink/Logic and Bit Operations/Compare To Constant  SystemSampleTime=-1  relop=<=  const=59.8  LogicOutDataTypeMode=boolean
  Compare To Constant2 : simulink/Logic and Bit Operations/Compare To Constant  SystemSampleTime=-1  relop=<=  const=59.5  LogicOutDataTypeMode=boolean
  Compare To Constant3 : simulink/Logic and Bit Operations/Compare To Constant  SystemSampleTime=-1  relop=>=  const=59.9  LogicOutDataTypeMode=boolean
  Compare To Constant4 : simulink/Logic and Bit Operations/Compare To Constant  SystemSampleTime=-1  relop=<=  const=58.6  LogicOutDataTypeMode=boolean
  Compare To Constant5 : simulink/Logic and Bit Operations/Compare To Constant  SystemSampleTime=-1  relop=<=  const=100  LogicOutDataTypeMode=boolean
  Mux : Mux
  "RMS " : powerlib_extras/Measurements/RMS  DialogController=POWERSYS.PowerSysDialog  SystemSampleTime=-1  f1=60
  RMS1 : powerlib_extras/Measurements/RMS  DialogController=POWERSYS.PowerSysDialog  SystemSampleTime=-1  f1=60
  frequency estimator (discrete) : Subsystem  mask{dt=0.010}
      mask prompts: dt "sample time"
  load shedding logic : M-S-Function  FunctionName=load_shedding_logic  Parameters=p
  w : Outport  OutDataType=fixdt(1, 16)  OutScaling=2^0
  trip : Outport  Port=2
  Irms : Outport  Port=3  OutDataType=fixdt(1, 16)  OutScaling=2^0
  Vrms : Outport  Port=4  OutDataType=fixdt(1, 16)  OutScaling=2^0
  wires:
  "RMS "/1 -> Compare To Constant/1, Irms/1
  I/1 -> "RMS "/1
  Reset/1 -> load shedding logic/1
  Compare To Constant/1 -> load shedding logic/2
  load shedding logic/1 -> trip/1
  V/1 -> frequency estimator (discrete)/1(v), RMS1/1
  frequency estimator (discrete)/1(w) -> Compare To Constant1/1, w/1, Compare To Constant2/1, Compare To Constant3/1, Compare To Constant4/1
  Compare To Constant1/1 -> Mux/1
  Compare To Constant2/1 -> Mux/2
  Compare To Constant3/1 -> Mux/3
  Compare To Constant4/1 -> Mux/4
  RMS1/1 -> Compare To Constant5/1, Vrms/1
  Compare To Constant5/1 -> load shedding logic/3
  Mux/1 -> load shedding logic/4

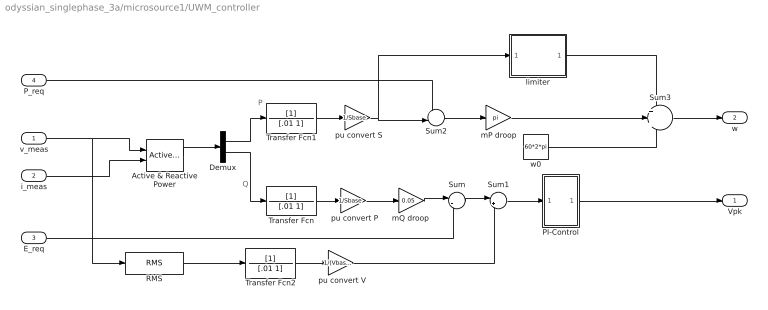
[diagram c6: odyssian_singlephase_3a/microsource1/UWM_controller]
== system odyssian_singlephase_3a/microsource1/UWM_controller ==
  note: P
  note: Q
  v_meas : Inport
  i_meas : Inport  Port=2
  E_req : Inport  Port=3
  P_req : Inport  Port=4
  " pu convert P" : Gain  Gain=1/Sbase  ParameterDataType=sfix(16)  ParameterScaling=2^0  OutDataType=sfix(16)  OutScaling=2^0
  " pu convert S" : Gain  Gain=1/Sbase  ParameterDataType=sfix(16)  ParameterScaling=2^0  OutDataType=sfix(16)  OutScaling=2^0
  " pu convert V" : Gain  Gain=1/(Vbase/sqrt(2))  ParameterDataType=sfix(16)  ParameterScaling=2^0  OutDataType=sfix(16)  OutScaling=2^0
  Active & Reactive Power : powerlib_extras/Measurements/Active & Reactive Power  DialogController=POWERSYS.PowerSysDialog  SystemSampleTime=-1  f1=60
  Demux : Demux  Outputs=2
  PI-Control : Subsystem
  RMS : powerlib_extras/Measurements/RMS  DialogController=POWERSYS.PowerSysDialog  SystemSampleTime=-1  f1=60
  Sum : Sum  Inputs=|-+  OutDataType=sfix(16)  OutScaling=2^0
  Sum1 : Sum  Inputs=|+-  OutDataType=sfix(16)  OutScaling=2^0
  Sum2 : Sum  Inputs=+-|  OutDataType=sfix(16)  OutScaling=2^0
  Sum3 : Sum  Inputs=+++  OutDataType=sfix(16)  OutScaling=2^0
  Transfer Fcn : TransferFcn  Denominator=[.01 1]
  Transfer Fcn1 : TransferFcn  Denominator=[.01 1]
  Transfer Fcn2 : TransferFcn  Denominator=[.01 1]
  limiter : Subsystem
  mP droop : Gain  Gain=pi  ParameterDataType=sfix(16)  ParameterScaling=2^0  OutDataType=sfix(16)  OutScaling=2^0
  "mQ droop " : Gain  Gain=0.05  ParameterDataType=sfix(16)  ParameterScaling=2^0  OutDataType=sfix(16)  OutScaling=2^0
  w0 : Constant  Value=60*2*pi  OutDataType=fixdt(1, 16)  OutScaling=2^0
  Vpk : Outport
  w : Outport  Port=2
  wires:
  Transfer Fcn2/1 -> " pu convert V"/1
  Transfer Fcn/1 -> " pu convert P"/1
  " pu convert P"/1 -> "mQ droop "/1
  Transfer Fcn1/1 -> " pu convert S"/1
  " pu convert S"/1 -> limiter/1(In1), Sum2/2
  i_meas/1 -> Active & Reactive Power/2
  P_req/1 -> Sum2/1
  mP droop/1 -> Sum3/2
  limiter/1(Out1) -> Sum3/1
  w0/1 -> Sum3/3
  Sum2/1 -> mP droop/1
  Sum1/1 -> PI-Control/1(In1)
  Sum/1 -> Sum1/1
  "mQ droop "/1 -> Sum/1
  Demux/2 -> Transfer Fcn/1
  Demux/1 -> Transfer Fcn1/1
  Active & Reactive Power/1 -> Demux/1
  v_meas/1 -> RMS/1, Active & Reactive Power/1
  PI-Control/1(Out1) -> Vpk/1
  Sum3/1 -> w/1
  E_req/1 -> Sum/2
  " pu convert V"/1 -> Sum1/2
  RMS/1 -> Transfer Fcn2/1

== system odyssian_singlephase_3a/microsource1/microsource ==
  Vpk : Inport  OutDataType=fixdt(1, 16)  OutScaling=2^0
  w : Inport  Port=2  OutDataType=fixdt(1, 16)  OutScaling=2^0
  Integrator : Integrator
  Product : Product  OutDataType=sfix(16)  OutScaling=2^0
  phaseA : powerlib/Electrical Sources/Controlled Voltage Source  DialogController=POWERSYS.PowerSysDialog  SystemSampleTime=-1  Initialize=on  Source_Type=AC  Amplitude=0  Phase=0  Frequency=0  Measurements=None
  v_A : Fcn  Expr=cos(u)
  Va : PMIOPort  Tag=PMCPort  Port=1  Side=Right
  Neutral : PMIOPort  Tag=PMCPort  Port=2  Side=Right
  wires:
  Product/1 -> phaseA/1
  Vpk/1 -> Product/1
  w/1 -> Integrator/1
  Integrator/1 -> v_A/1
  v_A/1 -> Product/2
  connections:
  phaseA/RConn1 -- Va/RConn1
  phaseA/LConn1 -- Neutral/RConn1

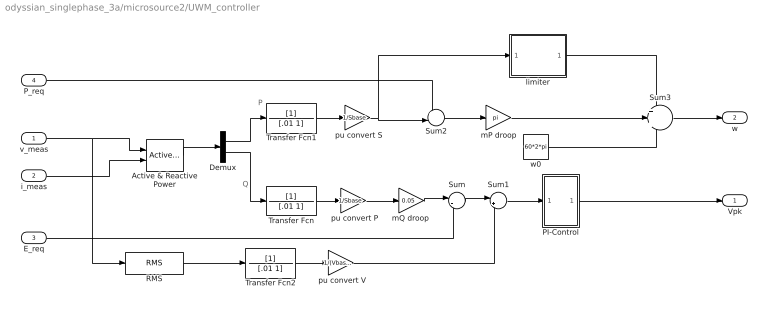
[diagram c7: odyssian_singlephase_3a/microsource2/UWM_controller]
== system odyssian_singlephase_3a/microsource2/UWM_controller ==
  note: P
  note: Q
  v_meas : Inport
  i_meas : Inport  Port=2
  E_req : Inport  Port=3
  P_req : Inport  Port=4
  " pu convert P" : Gain  Gain=1/Sbase  ParameterDataType=sfix(16)  ParameterScaling=2^0  OutDataType=sfix(16)  OutScaling=2^0
  " pu convert S" : Gain  Gain=1/Sbase  ParameterDataType=sfix(16)  ParameterScaling=2^0  OutDataType=sfix(16)  OutScaling=2^0
  " pu convert V" : Gain  Gain=1/(Vbase/sqrt(2))  ParameterDataType=sfix(16)  ParameterScaling=2^0  OutDataType=sfix(16)  OutScaling=2^0
  Active & Reactive Power : powerlib_extras/Measurements/Active & Reactive Power  DialogController=POWERSYS.PowerSysDialog  SystemSampleTime=-1  f1=60
  Demux : Demux  Outputs=2
  PI-Control : Subsystem
  RMS : powerlib_extras/Measurements/RMS  DialogController=POWERSYS.PowerSysDialog  SystemSampleTime=-1  f1=60
  Sum : Sum  Inputs=|-+  OutDataType=sfix(16)  OutScaling=2^0
  Sum1 : Sum  Inputs=|+-  OutDataType=sfix(16)  OutScaling=2^0
  Sum2 : Sum  Inputs=+-|  OutDataType=sfix(16)  OutScaling=2^0
  Sum3 : Sum  Inputs=+++  OutDataType=sfix(16)  OutScaling=2^0
  Transfer Fcn : TransferFcn  Denominator=[.01 1]
  Transfer Fcn1 : TransferFcn  Denominator=[.01 1]
  Transfer Fcn2 : TransferFcn  Denominator=[.01 1]
  limiter : Subsystem
  mP droop : Gain  Gain=pi  ParameterDataType=sfix(16)  ParameterScaling=2^0  OutDataType=sfix(16)  OutScaling=2^0
  "mQ droop " : Gain  Gain=0.05  ParameterDataType=sfix(16)  ParameterScaling=2^0  OutDataType=sfix(16)  OutScaling=2^0
  w0 : Constant  Value=60*2*pi  OutDataType=fixdt(1, 16)  OutScaling=2^0
  Vpk : Outport
  w : Outport  Port=2
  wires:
  Transfer Fcn2/1 -> " pu convert V"/1
  Transfer Fcn/1 -> " pu convert P"/1
  " pu convert P"/1 -> "mQ droop "/1
  Transfer Fcn1/1 -> " pu convert S"/1
  " pu convert S"/1 -> limiter/1(In1), Sum2/2
  i_meas/1 -> Active & Reactive Power/2
  P_req/1 -> Sum2/1
  mP droop/1 -> Sum3/2
  limiter/1(Out1) -> Sum3/1
  w0/1 -> Sum3/3
  Sum2/1 -> mP droop/1
  Sum1/1 -> PI-Control/1(In1)
  Sum/1 -> Sum1/1
  "mQ droop "/1 -> Sum/1
  Demux/2 -> Transfer Fcn/1
  Demux/1 -> Transfer Fcn1/1
  Active & Reactive Power/1 -> Demux/1
  v_meas/1 -> RMS/1, Active & Reactive Power/1
  PI-Control/1(Out1) -> Vpk/1
  Sum3/1 -> w/1
  E_req/1 -> Sum/2
  " pu convert V"/1 -> Sum1/2
  RMS/1 -> Transfer Fcn2/1

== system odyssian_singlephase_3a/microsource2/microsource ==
  Vpk : Inport  OutDataType=fixdt(1, 16)  OutScaling=2^0
  w : Inport  Port=2  OutDataType=fixdt(1, 16)  OutScaling=2^0
  Integrator : Integrator
  Product : Product  OutDataType=sfix(16)  OutScaling=2^0
  phaseA : powerlib/Electrical Sources/Controlled Voltage Source  DialogController=POWERSYS.PowerSysDialog  SystemSampleTime=-1  Initialize=on  Source_Type=AC  Amplitude=0  Phase=0  Frequency=0  Measurements=None
  v_A : Fcn  Expr=cos(u)
  Va : PMIOPort  Tag=PMCPort  Port=1  Side=Right
  Neutral : PMIOPort  Tag=PMCPort  Port=2  Side=Right
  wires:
  Product/1 -> phaseA/1
  Vpk/1 -> Product/1
  w/1 -> Integrator/1
  Integrator/1 -> v_A/1
  v_A/1 -> Product/2
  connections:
  phaseA/RConn1 -- Va/RConn1
  phaseA/LConn1 -- Neutral/RConn1
